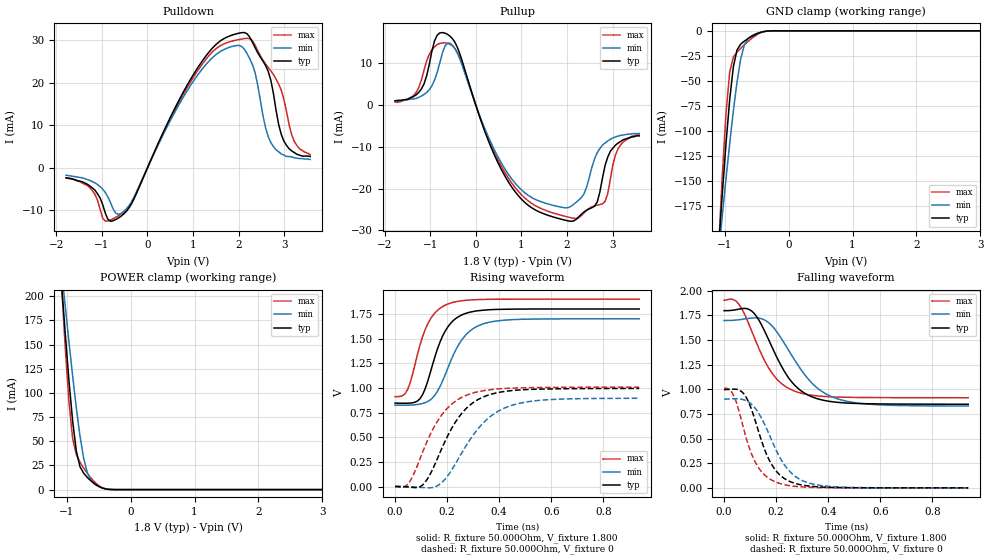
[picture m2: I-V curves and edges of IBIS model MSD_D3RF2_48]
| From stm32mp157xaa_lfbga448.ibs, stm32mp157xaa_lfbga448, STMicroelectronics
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[Model] MSD_D3RF2_48
Model_type   I/O
C_comp 2.228pF   2.149pF   2.345pF
Vinh = 1.150V
Vinl = 650.000mV
Vmeas = 900.000mV
Vref = 900.000mV
[Model Spec]
Vinh   1.150V   1.100V   1.200V
Vinl   650.000mV   600.000mV   700.000mV
Vmeas   900.000mV   850.000mV   950.000mV
Vref   900.000mV   850.000mV   950.000mV
[Temperature Range]   25.000   125.000   -40.000
[Voltage Range]   1.800V   1.700V   1.900V
[GND Clamp Reference]   0.00V   0.00V   0.00V
[Pulldown Reference]   0.00V   0.00V   0.00V
[POWER Clamp Reference]   1.800V   1.700V   1.900V
[Pullup Reference]   1.800V   1.700V   1.900V
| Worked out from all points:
|   slope of the pulldown table from 0 to 0.27 V, typ, clamps not added: 41 ohm
|   slope of the pullup table from 0 to 0.27 V, typ, clamps not added: 32.3 ohm
|   GND clamp passes 1 mA (typ) near -0.41 V on its own axis
|   POWER clamp passes 1 mA (typ) near -0.41 V on its own axis
|   rising waveform, R_fixture 50.000Ohm, V_fixture 1.800: 20-80 % time 79.1ps typ, 98.1ps min, 72.7ps max; typ from 0.846 V to 1.8 V
|   rising waveform, R_fixture 50.000Ohm, V_fixture 0: 20-80 % time 126ps typ, 149ps min, 121ps max; typ from 0.001 V to 0.994 V
|   falling waveform, R_fixture 50.000Ohm, V_fixture 1.800: 20-80 % time 120ps typ, 145ps min, 112ps max; typ from 1.8 V to 0.849 V
|   falling waveform, R_fixture 50.000Ohm, V_fixture 0: 20-80 % time 86.7ps typ, 107ps min, 79.1ps max; typ from 0.997 V to 0 V
[GND Clamp]
-1.785V   -901.2mA   -688.7mA   -1.21A
-1.094V   -214.6mA   -220.9mA   -215.3mA
-1.036V   -161.8mA   -183.6mA   -143.3mA
-978.8mV  -112.2mA   -147.3mA   -82mA
-921.2mV  -68.48mA   -112.3mA   -40.93mA
-863.6mV  -35.72mA   -79.61mA   -26.14mA
-806.1mV  -18.98mA   -50.61mA   -21.24mA
-748.5mV  -13.21mA   -27.8mA    -17.43mA
-690.9mV  -10.21mA   -13.79mA   -13.87mA
-575.8mV  -5.519mA   -4.737mA   -7.464mA
-287.9mV  -70.53uA   -119uA     -55.71uA
3.57V     33.94nA    572.8nA    3.717nA
[Power Clamp]
-1.77V    882.6mA    689.8mA    1.159A
-1.079V   212.4mA    226.5mA    212.1mA
-1.021V   160.9mA    189.3mA    146.7mA
-963.6mV  112.9mA    152.9mA    90.89mA
-906.1mV  71.15mA    117.8mA    52.89mA
-848.5mV  40.01mA    84.75mA    36.15mA
-790.9mV  23.77mA    55.41mA    28.47mA
-733.3mV  16.96mA    32.2mA     22.3mA
-618.2mV  8.941mA    9.722mA    11.92mA
-503mV    3.409mA    3.507mA    4.442mA
-272.7mV  29.94uA    100.2uA    29.64uA
3.585V    -51.59nA   -929.3nA   -5.523nA
[Pulldown]
-1.785V   -2.3mA     -1.7mA     -2.4mA
-1.267V   -4.2mA     -2.9mA     -4.6mA
-921.2mV  -10.71mA   -5.8mA     -12.53mA
-575.8mV  -11.32mA   -10.68mA   -10.83mA
1.094V    23.43mA    21.74mA    22.76mA
1.612V    29.99mA    27.49mA    28.84mA
2.073V    31.84mA    28.54mA    30.34mA
2.361V    28.32mA    22.42mA    28.91mA
2.706V    20.69mA    6mA        22.85mA
2.994V    6.3mA      3mA        16.1mA
3.224V    3.6mA      2.4mA      6.2mA
3.57V     2.7mA      2mA        3.1mA
[Pullup]
-1.77V    1mA        900uA      673.7uA
-1.309V   2.4mA      1.547mA    2.963mA
-1.021V   9.6mA      3.616mA    12.09mA
-848.5mV  16.65mA    7.7mA      14.42mA
-618.2mV  16.89mA    14.81mA    14.74mA
763.6mV   -19.22mA   -17.32mA   -18.27mA
2.088V    -27.84mA   -24.27mA   -26.98mA
2.376V    -25.59mA   -21.23mA   -25.8mA
2.606V    -24.21mA   -12.89mA   -24.14mA
2.779V    -17.5mA    -9.61mA    -23.66mA
3.124V    -9.1mA     -7.453mA   -10.44mA
3.585V    -7.4mA     -6.826mA   -7.047mA
[Ramp]
R_load=50.000Ohm
dV/dt_r   583.800mV/103.000ps  529.889mV/124.500ps  597.810mV/97.500ps
dV/dt_f   583.800mV/104.500ps  529.889mV/126.500ps  597.810mV/96.500ps
[Rising waveform]
R_fixture=50.000Ohm
V_fixture=1.800
V_fixture_min=1.700
V_fixture_max=1.900
0s        845.6mV    824.6mV    911.1mV
29ps      844.1mV    823.9mV    920.8mV
48ps      844.4mV    824.5mV    981.5mV
96ps      891.1mV    836.2mV    1.437V
135ps     1.151V     877.6mV    1.695V
173ps     1.467V     1.015V     1.808V
202ps     1.615V     1.195V     1.85V
259ps     1.743V     1.497V     1.884V
345ps     1.789V     1.655V     1.897V
938ps     1.8V       1.7V       1.9V
[Rising waveform]
R_fixture=50.000Ohm
V_fixture=0
0s        667uV      601.1uV    -2.314mV
48ps      -4.293mV   -1.405mV   19.81mV
87ps      -10.12mV   -6.693mV   220.1mV
115ps     41.69mV    -12.41mV   407.6mV
183ps     406.2mV    48.7mV     738.6mV
230ps     645.1mV    221.8mV    860.9mV
269ps     779.8mV    396.8mV    919.9mV
355ps     923.9mV    685.6mV    978.1mV
460ps     975.3mV    831.7mV    998.5mV
938ps     994.2mV    894.6mV    1.007V
[Falling waveform]
R_fixture=50.000Ohm
V_fixture=1.800
V_fixture_min=1.700
V_fixture_max=1.900
0s        1.799V     1.699V     1.904V
29ps      1.802V     1.7V       1.916V
58ps      1.815V     1.707V     1.86V
115ps     1.773V     1.726V     1.534V
183ps     1.436V     1.648V     1.17V
269ps     1.048V     1.307V     984mV
355ps     907.4mV    1.02V      934.6mV
441ps     867mV      899.2mV    921.2mV
595ps     852.2mV    843mV      916.5mV
938ps     848.7mV    830.6mV    914.9mV
[Falling waveform]
R_fixture=50.000Ohm
V_fixture=0
0s        996.7mV    899.8mV    1.013V
39ps      1.002V     905mV      925.7mV
87ps      910.4mV    882.7mV    488.5mV
106ps     792.6mV    846.9mV    341.3mV
135ps     550.7mV    749mV      194.4mV
163ps     341mV      603.8mV    114.2mV
202ps     164.7mV    371.5mV    55.59mV
269ps     48.55mV    125.2mV    16.63mV
355ps     11.58mV    31.22mV    3.614mV
938ps     14.81uV    27.75uV    -1.489uV
